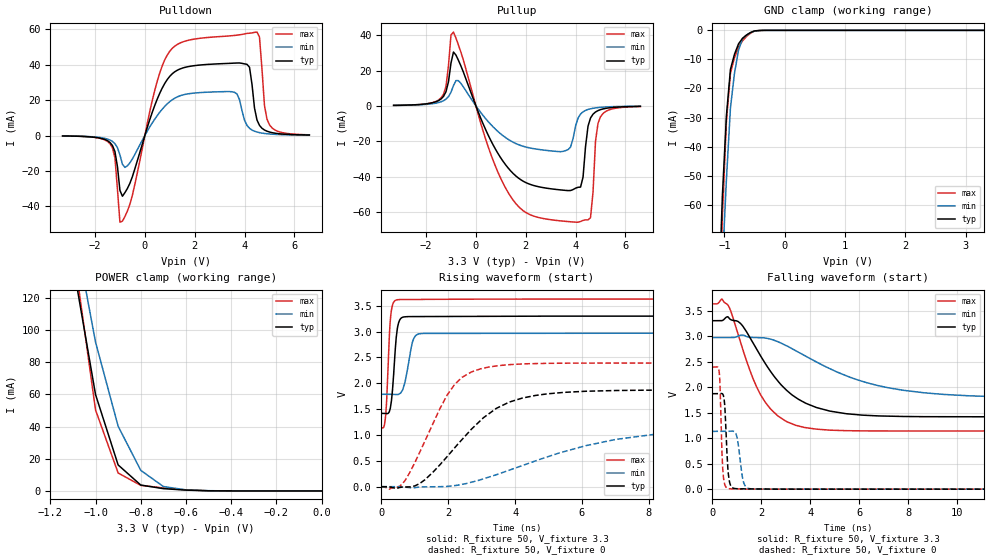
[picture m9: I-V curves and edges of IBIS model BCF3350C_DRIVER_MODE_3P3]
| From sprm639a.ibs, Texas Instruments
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|   Model Cell BCF3350C_DRIVER_MODE_3P3
|BCF3350C_DRIVER_MODE_3P3
[Model]   BCF3350C_DRIVER_MODE_3P3
Model_type   I/O
Polarity   Non-Inverting
Enable   Active-Low
Vinl =  0.8
Vinh =  2
Cref =  15.0000pF
Rref =  100.0000M
Vref =  0V
Vmeas =  1.65
C_comp   1.081618p   0.946736p   1.221412p
[Model Spec]
Vinl   0.8   0.8   0.8
Vinh   2   2   2
[Temperature Range]   25   155   -40
[Voltage Range]   3.3   2.97   3.63
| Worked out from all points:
|   slope of the pulldown table from 0 to 0.495 V, typ, clamps not added: 24.2 ohm
|   slope of the pullup table from 0 to 0.495 V, typ, clamps not added: 29.8 ohm
|   GND clamp passes 1 mA (typ) near -0.59 V on its own axis
|   POWER clamp passes 1 mA (typ) near -0.65 V on its own axis
|   rising waveform, R_fixture 50, V_fixture 3.3: 20-80 % time 128ps typ, 199ps min, 103ps max; typ from 1.42 V to 3.3 V
|   rising waveform, R_fixture 50, V_fixture 0: 20-80 % time 1.72ns typ, 3.53ns min, 1.11ns max; typ from 0 V to 1.87 V
|   falling waveform, R_fixture 50, V_fixture 3.3: 20-80 % time 1.82ns typ, 3.49ns min, 1.28ns max; typ from 3.3 V to 1.42 V
|   falling waveform, R_fixture 50, V_fixture 0: 20-80 % time 116ps typ, 184ps min, 93.4ps max; typ from 1.87 V to 0 V
| Nom Voltages:
|   VDD=1.2, VDDS=3.3, VSS=0
| Min Voltages:
|   VDD=1.08, VDDS=2.97, VSS=0
| Max Voltages:
|   VDD=1.32, VDDS=3.63, VSS=0
[POWER_clamp]
|   voltage   I(typ)   I(min)   I(max)
-3.3V     2.318A     2.595A     3.049A
-1.1V     141.5mA    168mA      152.3mA
-1.067V   114.3mA    142.9mA    118.3mA
-1.033V   87.17mA    117.8mA    84.37mA
-1V       60.01mA    92.63mA    50.4mA
-900mV    16.17mA    40.25mA    11.16mA
-800mV    3.655mA    12.81mA    3.461mA
-700mV    1.415mA    2.754mA    1.844mA
-600mV    504.3uA    641.1uA    658.2uA
-500mV    86.55uA    148.2uA    94.22uA
0V        39.59pA    2.724nA    9.668pA
[Pulldown]
|   voltage   I(typ)   I(min)   I(max)
-3.3V     -252.1uA   -234.7uA   -277.7uA
-1.4V     -3.919mA   -2.547mA   -4.608mA
-1.2V     -9.103mA   -4.609mA   -12.64mA
-900mV    -34.3mA    -16.21mA   -48.36mA
1V        33.43mA    19.12mA    47.58mA
3.6V      40.87mA    24.35mA    56.5mA
4.1V      40.18mA    5.681mA    57.63mA
4.5V      8.744mA    1.956mA    58.39mA
4.6V      5.703mA    1.616mA    55.56mA
4.8V      3.099mA    1.152mA    16.91mA
5V        1.969mA    859.8uA    6.049mA
6.6V      281.1uA    214.2uA    387.2uA
[Pullup]
|   voltage   I(typ)   I(min)   I(max)
-3.3V     278.9uA    242.8uA    252.3uA
-1.4V     3.885mA    2.29mA     4.485mA
-900mV    30.46mA    11.45mA    41.76mA
500mV     -16.76mA   -9.024mA   -23.45mA
1.4V      -36.9mA    -19.86mA   -51.44mA
3.6V      -47.86mA   -25.33mA   -65.39mA
4.1V      -46.11mA   -6.928mA   -65.87mA
4.3V      -40.29mA   -3.368mA   -64.88mA
4.6V      -6.878mA   -1.656mA   -63.29mA
4.8V      -3.477mA   -1.154mA   -20.01mA
5V        -2.143mA   -846.4uA   -6.19mA
6.6V      -290.9uA   -205.6uA   -395.4uA
[GND_clamp]
|   voltage   I(typ)   I(min)   I(max)
-3.3V     -1.888A    -1.585A    -3.154A
-1.1V     -95.78mA   -113.9mA   -112.1mA
-1.033V   -56.7mA    -80.3mA    -63.61mA
-966.7mV  -29.24mA   -51.23mA   -31.16mA
-900mV    -13.41mA   -26.67mA   -14.73mA
-833.3mV  -8.233mA   -14.78mA   -9.457mA
-766.7mV  -4.676mA   -6.859mA   -5.761mA
-700mV    -2.737mA   -2.908mA   -3.644mA
-566.7mV  -742.7uA   -781uA     -966.3uA
-500mV    -188.9uA   -280.3uA   -215.5uA
-366.7mV  -8.774uA   -27.7uA    -8.181uA
3.3V      39.59pA    4.205uA    5.4pA
[Ramp]
| variable   typ   min   max
dV/dt_f  1.1758078/1.8487904n 0.73903787/3.5515044n   1.550806/1.2968051n
dV/dt_r  1.1447184/1.7447243n 0.69386454/3.5889294n  1.4638499/1.1276797n
R_load = 50
[Rising Waveform]
R_fixture = 50
V_fixture = 3.3
V_fixture_min = 2.97
V_fixture_max = 3.63
|   time   V(typ)   V(min)   V(max)
0s        1.419V     1.788V     1.14V
82.3ps    1.418V     1.788V     1.168V
134.6ps   1.416V     1.788V     1.414V
267.9ps   1.514V     1.788V     3.209V
334.7ps   1.872V     1.787V     3.516V
476ps     3.044V     1.783V     3.617V
710.4ps   3.287V     2.026V     3.621V
975.3ps   3.291V     2.875V     3.62V
1.167ns   3.292V     2.962V     3.623V
20.01ns   3.3V       2.97V      3.63V
[Rising Waveform]
R_fixture = 50
V_fixture = 0
V_fixture_min = 0
V_fixture_max = 0
|   time   V(typ)   V(min)   V(max)
0s        0V         0V         0V
633.9ps   -7.963mV   -4.754mV   56.74mV
1.147ns   60.6mV     -6.563mV   662.7mV
1.744ns   417.8mV    0V         1.5V
2.192ns   750.8mV    20.94mV    1.979V
3.241ns   1.422V     190.2mV    2.319V
4.598ns   1.764V     497.4mV    2.382V
6.086ns   1.845V     790.2mV    2.391V
8.217ns   1.868V     1.017V     2.392V
20.06ns   1.87V      1.132V     2.392V
[Falling Waveform]
R_fixture = 50
V_fixture = 3.3
V_fixture_min = 2.97
V_fixture_max = 3.63
|   time   V(typ)   V(min)   V(max)
0s        3.3V       2.97V      3.63V
383.9ps   3.301V     2.97V      3.724V
646.9ps   3.371V     2.97V      3.6V
1.142ns   3.252V     3.015V     2.893V
1.667ns   2.861V     2.972V     2.161V
2.148ns   2.472V     2.961V     1.711V
3.398ns   1.799V     2.715V     1.252V
5.976ns   1.457V     2.134V     1.142V
8.624ns   1.42V      1.889V     1.14V
20.01ns   1.419V     1.788V     1.14V
[Falling Waveform]
R_fixture = 50
V_fixture = 0
V_fixture_min = 0
V_fixture_max = 0
|   time   V(typ)   V(min)   V(max)
0s        1.87V      1.132V     2.392V
282.4ps   1.871V     1.132V     2.285V
388.8ps   1.874V     1.132V     759.4mV
449.9ps   1.838V     1.132V     250.1mV
518.2ps   1.545V     1.132V     72.7mV
627.8ps   445.1mV    1.133V     13.65mV
955.9ps   10.3mV     1.094V     6.134mV
1.278ns   6.846mV    130.4mV    2.477mV
1.549ns   5.09mV     7.584mV    0V
20.06ns   0V         0V         0V
